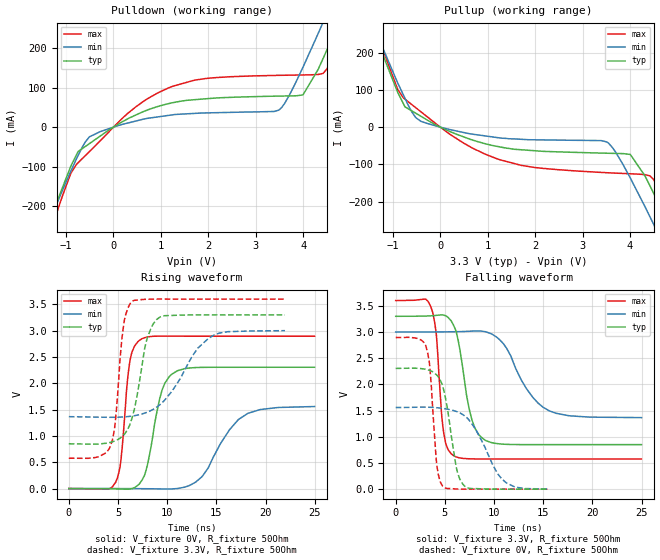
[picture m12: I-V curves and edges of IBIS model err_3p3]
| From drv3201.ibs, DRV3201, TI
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|   err_3p3 Model
[Model]   err_3p3
Model_type   Output
Polarity   Non-Inverting
Vmeas = 1.65
Vref = 0
Cref = 2pF
Rref = 300
|   typ   min   max
|   (nom PVT)   (fast PVT)   (slow PVT)
 C_comp   3.809e-12   3.780e-12   4.057e-12
| Where nom  PVT is Nominal Process, 3.3V, 27C
|   Fast PVT is Strong Process,  3.6V, -40C
|   Slow PVT is Weak Process,   3V, 150C
[Voltage Range]   3.3   3   3.6
|Junction Temperature
[Temperature Range]   27   150   -40
[Pullup Reference]   3.3   3   3.6
[Pulldown Reference]   0   0   0
[Power Clamp Reference]   3.3   3   3.6
[GND Clamp Reference]   0   0   0
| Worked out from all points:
|   slope of the pulldown table from 0 to 0.495 V, typ, clamps not added: 15.5 ohm
|   slope of the pullup table from 0 to 0.495 V, typ, clamps not added: 18.8 ohm
|   falling waveform, V_fixture 3.3V, R_fixture 50Ohm: 20-80 % time 1.34ns typ, 2.91ns min, 700ps max; typ from 3.3 V to 0.85 V
|   rising waveform, V_fixture 0V, R_fixture 50Ohm: 20-80 % time 1.43ns typ, 3.07ns min, 810ps max; typ from 0 V to 2.31 V
|   rising waveform, V_fixture 3.3V, R_fixture 50Ohm: 20-80 % time 1.47ns typ, 3.34ns min, 824ps max; typ from 0.85 V to 3.3 V
|   falling waveform, V_fixture 0V, R_fixture 50Ohm: 20-80 % time 1.17ns typ, 2.57ns min, 638ps max; typ from 2.31 V to 0 V
[Pulldown]
|   Voltage   I(typ)   I(min)   I(max)
-3.3V     -890.9mA   -821.6mA   -986.4mA
-1.458V   -274.2mA   -268.7mA   -310mA
-1.238V   -202.6mA   -205.8mA   -231.5mA
-745.8mV  -61.74mA   -71.93mA   -89.89mA
-507mV    -41.71mA   -24.53mA   -61.92mA
1.174V    59.69mA    29.88mA    99.8mA
3.486V    78.44mA    43.02mA    130.9mA
3.996V    81.47mA    151.6mA    131.9mA
4.421V    173.7mA    265.3mA    135.8mA
4.795V    279.6mA    371.5mA    223.1mA
5.303V    425.2mA    516.9mA    372.4mA
6.6V      822.4mA    888.5mA    785.1mA
[Pullup]
|   Voltage   I(typ)   I(min)   I(max)
-3.3V     887.3mA    853.6mA    954.6mA
-1.39V    251.2mA    264.8mA    268.2mA
-896.4mV  92.89mA    117.9mA    100.5mA
-745.8mV  54.5mA     77.5mA     75.07mA
-516mV    37.19mA    25.33mA    51.94mA
939.6mV   -44.29mA   -23.44mA   -72.13mA
3.51V     -69.95mA   -39.73mA   -122.3mA
4.006V    -73.26mA   -136.5mA   -125.1mA
4.507V    -180mA     -263.2mA   -142.4mA
4.813V    -267.2mA   -345.9mA   -221.1mA
5.205V    -378.9mA   -451.8mA   -338.5mA
6.6V      -809.2mA   -849.2mA   -796.9mA
[Ramp]
R_load = 50
|   typ   min   max
dV/dt_r   1.38285/1.42488e-09   0.934955/2.99859e-09   1.73702/8.08205e-10
dV/dt_f   1.46991/1.33597e-09   0.980652/2.8878e-09   1.81426/6.94982e-10
[Falling Waveform]
V_fixture = 3.3V
V_fixture_min = 3V
V_fixture_max = 3.6V
R_fixture = 50Ohm
|   Time   V(typ)   V(min)   V(max)
0s        3.3V       3V         3.6V
3.576ns   3.309V     3.001V     3.481V
4.114ns   3.317V     3.002V     2.986V
4.884ns   3.322V     3.003V     1.071V
5.884ns   3.128V     3.005V     641mV
7.744ns   1.325V     3.017V     578.2mV
9.116ns   931.9mV    3.006V     576mV
10.96ns   858.5mV    2.774V     576.2mV
15.61ns   850.1mV    1.496V     576.2mV
24.98ns   850.1mV    1.366V     576.2mV
[Rising Waveform]
V_fixture = 0V
V_fixture_min = 0V
V_fixture_max = 0V
R_fixture = 50Ohm
|   Time   V(typ)   V(min)   V(max)
0s        522.1pV    191.1nV    366.5pV
4.75ns    -5.471mV   -234uV     114.6mV
5.306ns   -8.591mV   -596.2uV   553.4mV
6.25ns    -7.908mV   -1.475mV   2.461V
7.426ns   154.7mV    -2.981mV   2.846V
9.492ns   1.877V     -7.595mV   2.896V
10.46ns   2.172V     -7.599mV   2.896V
13.5ns    2.302V     217.9mV    2.895V
18.21ns   2.305V     1.429V     2.895V
24.99ns   2.305V     1.558V     2.895V
[Rising Waveform]
V_fixture = 3.3V
V_fixture_min = 3V
V_fixture_max = 3.6V
R_fixture = 50Ohm
|   Time   V(typ)   V(min)   V(max)
0s        850.1mV    1.366V     576.2mV
4.234ns   878.1mV    1.354V     809.5mV
4.754ns   910.5mV    1.355V     1.319V
5.248ns   962.3mV    1.358V     2.548V
5.576ns   1.016V     1.361V     3.112V
6.42ns    1.335V     1.377V     3.555V
7.968ns   2.856V     1.451V     3.597V
9.252ns   3.257V     1.592V     3.601V
14.74ns   3.3V       2.914V     3.6V
21.98ns   3.3V       3V         3.6V
[Falling Waveform]
V_fixture = 0V
V_fixture_min = 0V
V_fixture_max = 0V
R_fixture = 50Ohm
|   Time   V(typ)   V(min)   V(max)
0s        2.305V     1.558V     2.895V
3.088ns   2.286V     1.565V     2.721V
3.508ns   2.262V     1.563V     2.247V
4.204ns   2.174V     1.554V     423.6mV
4.782ns   1.963V     1.542V     54.87mV
5.21ns    1.588V     1.529V     14.75mV
6.14ns    430.7mV    1.485V     3.844mV
7.018ns   56.11mV    1.398V     690.4uV
10.8ns    285.1uV    193.7mV    -4.998uV
15.43ns   -736.3nV   3.175mV    -72.21nV
